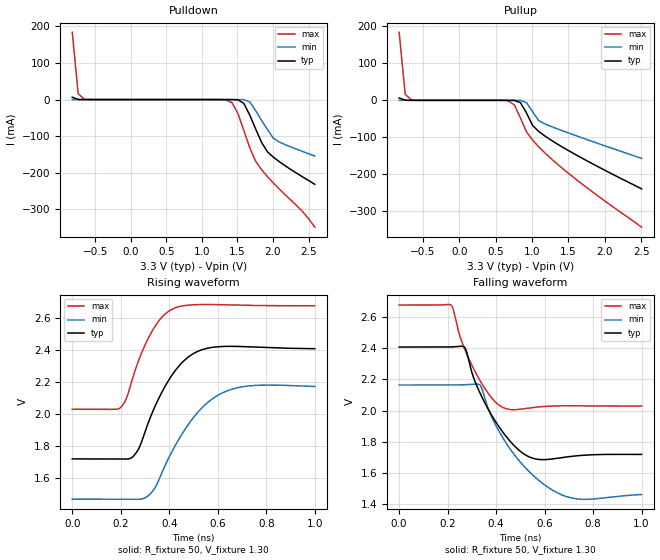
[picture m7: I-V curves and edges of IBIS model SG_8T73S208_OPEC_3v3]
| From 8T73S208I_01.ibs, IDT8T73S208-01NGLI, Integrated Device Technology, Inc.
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[Model] SG_8T73S208_OPEC_3v3
Model_type   Output_ECL
Polarity   Non-Inverting
|   typ   min   max
C_comp   2pF   1.5pF   2.5pF
Vmeas = 2.06V
Rref = 50
Cref = 0
Vref = 1.3V
|   typ   min   max
[Voltage range]   3.3V   3.135V   3.465V
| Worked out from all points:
|   rising waveform, R_fixture 50, V_fixture 1.30: 20-80 % time 131ps typ, 167ps min, 104ps max; typ from 1.72 V to 2.41 V
|   falling waveform, R_fixture 50, V_fixture 1.30: 20-80 % time 135ps typ, 176ps min, 108ps max; typ from 2.41 V to 1.72 V
[Pulldown]
|Voltage   I (typ)   I (min)   I (max)
|Note, modeling breaks down at 250mA and above.  This is well beyond the functional   |
|operating range of the device.  Should this scenario occur, catastrophic failure and   |
|possible damage to the device and/or board is of higher concern than the I-V curve   |
|behavior.  The IBIS checker will flag currents in excess of 10A with warnings.  Lines   |
|with currents in excess of 0.35 A have been commented out.  The points still remain|
|available to the user if the user desires to use them.   |
|-3.04000e+00   3.84320e+08   5.02796e+08   2.78359e+08
|-2.78000e+00   3.25714e+08   4.27850e+08   2.34472e+08
|-2.52000e+00   2.67107e+08   3.52905e+08   1.90585e+08
|-2.26000e+00   2.08500e+08   2.77959e+08   1.46698e+08
|-2.00000e+00   1.49893e+08   2.03013e+08   1.02811e+08
|-1.99000e+00   1.47639e+08   2.00131e+08   1.01123e+08
|-1.90678e+00   1.28880e+08   1.76142e+08   8.70758e+07
|-1.82356e+00   1.10121e+08   1.52153e+08   7.30282e+07
|-1.74033e+00   9.13618e+07   1.28164e+08   5.89806e+07
|-1.65711e+00   7.26027e+07   1.04175e+08   4.49331e+07
|-1.57389e+00   5.38435e+07   8.01855e+07   3.08855e+07
|-1.49067e+00   3.50844e+07   5.61965e+07   1.68379e+07
|-1.40744e+00   1.63252e+07   3.22075e+07   3.44928e+06
|-1.32422e+00   1.39944e+06   8.21842e+06   3.05002e+05
|-1.24100e+00   5.48675e+04   1.39917e+05   2.69841e+04
|-1.15778e+00   2.16294e+03   2.23572e+03   2.39776e+03
|-1.07456e+00   9.10504e+01   4.03625e+01   2.19447e+02
|-9.91333e-01   4.16516e+00   7.07425e-01   2.24205e+01
|-9.08111e-01   1.63247e-01   1.12381e-02   2.07885e+00
-824.9mV  6.398mA    178.5uA    183.8mA
-741.7mV  250.8uA    2.836uA    16.25mA
-658.4mV  9.828uA    45.07nA    1.437mA
1.256V    -48.99nA   -26.95pA   -86.69uA
1.422V    -28.87uA   -51.73nA   -8.139mA
1.505V    -675.9uA   -3.061uA   -37.65mA
1.589V    -10.23mA   -178.4uA   -83.91mA
1.672V    -41.96mA   -6.141mA   -131.5mA
1.755V    -80.08mA   -29.91mA   -168.3mA
1.921V    -142.8mA   -82.08mA   -210.6mA
2.005V    -157.3mA   -105.4mA   -228mA
2.587V    -231.4mA   -154.2mA   -348.7mA
| 2.67044e+00   -2.41524e-01   -1.60336e-01   -3.73288e-01
| 2.75367e+00   -2.52751e-01   -1.66631e-01   -3.98898e-01
| 2.83689e+00   -2.65451e-01   -1.73020e-01   -4.24212e-01
| 2.92011e+00   -2.79209e-01   -1.79583e-01   -4.49830e-01
| 3.00333e+00   -2.93544e-01   -1.86399e-01   -4.74213e-01
| 3.08656e+00   -3.07724e-01   -1.93355e-01   -4.94882e-01
| 3.16978e+00   -3.22002e-01   -2.00371e-01   -5.14267e-01
| 3.25300e+00   -3.36250e-01   -2.07556e-01   -5.33445e-01
| 3.33622e+00   -3.50790e-01   -2.15122e-01   -5.52591e-01
| 3.41944e+00   -3.64214e-01   -2.22630e-01   -5.71683e-01
| 3.50267e+00   -3.76611e-01   -2.29517e-01   -5.90648e-01
| 3.58589e+00   -3.88349e-01   -2.35518e-01   -6.09407e-01
| 3.66911e+00   -3.99917e-01   -2.41393e-01   -6.27633e-01
| 3.75233e+00   -4.11365e-01   -2.47762e-01   -6.44990e-01
| 3.83556e+00   -4.22795e-01   -2.54787e-01   -6.61715e-01
| 3.91878e+00   -4.34231e-01   -2.62348e-01   -6.78105e-01
| 4.00200e+00   -4.45476e-01   -2.70694e-01   -6.94450e-01
| 4.08522e+00   -4.57292e-01   -2.96778e-01   -7.11369e-01
| 4.16844e+00   -4.85300e-01   -3.52090e-01   -7.34921e-01
| 4.25167e+00   -5.33887e-01   -4.07605e-01   -7.78590e-01
| 4.33489e+00   -5.82604e-01   -4.63296e-01   -8.23081e-01
| 4.41811e+00   -6.31415e-01   -5.19140e-01   -8.67469e-01
| 4.50133e+00   -6.80294e-01   -5.75117e-01   -9.11758e-01
| 4.58456e+00   -7.29224e-01   -6.31213e-01   -9.55953e-01
| 4.66778e+00   -7.78192e-01   -6.87415e-01   -1.00006e+00
| 4.75100e+00   -8.27189e-01   -7.43713e-01   -1.04409e+00
| 4.83422e+00   -8.76208e-01   -8.00099e-01   -1.08807e+00
| 4.91744e+00   -9.25247e-01   -8.56569e-01   -1.13203e+00
| 5.00067e+00   -9.74313e-01   -9.13130e-01   -1.17598e+00
| 5.08389e+00   -1.02342e+00   -9.69776e-01   -1.21988e+00
| 5.16711e+00   -1.07255e+00   -1.02650e+00   -1.26381e+00
| 5.25033e+00   -1.12176e+00   -1.08332e+00   -1.30859e+00
| 5.33356e+00   -1.17164e+00   -1.14140e+00   -1.35828e+00
| 5.41678e+00   -1.22659e+00   -1.20480e+00   -1.40940e+00
| 5.50000e+00   -1.28295e+00   -1.26925e+00   -1.46042e+00
| 5.51000e+00   -1.28972e+00   -1.27702e+00   -1.46654e+00
| 5.72800e+00   -1.43794e+00   -1.44641e+00   -1.59960e+00
| 5.94600e+00   -1.59631e+00   -1.61583e+00   -1.73573e+00
| 6.16400e+00   -1.75745e+00   -1.78535e+00   -1.88508e+00
| 6.38200e+00   -1.91661e+00   -1.95502e+00   -2.03321e+00
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[Pullup]
|Voltage   I (typ)   I (min)   I (max)
|Note, modeling breaks down at 250mA and above.  This is well beyond the functional   |
|operating range of the device.  Should this scenario occur, catastrophic failure and   |
|possible damage to the device and/or board is of higher concern than the I-V curve   |
|behavior.  The IBIS checker will flag currents in excess of 10A with warnings.  Lines   |
|with currents in excess of 0.35 A have been commented out.  The points still remain|
|available to the user if the user desires to use them.   |
|-3.04000e+00   3.84320e+08   5.02796e+08   2.78359e+08
|-2.78000e+00   3.25714e+08   4.27850e+08   2.34472e+08
|-2.52000e+00   2.67107e+08   3.52905e+08   1.90585e+08
|-2.26000e+00   2.08500e+08   2.77959e+08   1.46698e+08
|-2.00000e+00   1.49893e+08   2.03013e+08   1.02811e+08
|-1.99000e+00   1.47639e+08   2.00131e+08   1.01123e+08
|-1.90678e+00   1.28880e+08   1.76142e+08   8.70758e+07
|-1.82356e+00   1.10121e+08   1.52153e+08   7.30282e+07
|-1.74033e+00   9.13618e+07   1.28164e+08   5.89806e+07
|-1.65711e+00   7.26027e+07   1.04175e+08   4.49331e+07
|-1.57389e+00   5.38435e+07   8.01855e+07   3.08855e+07
|-1.49067e+00   3.50844e+07   5.61965e+07   1.68379e+07
|-1.40744e+00   1.63252e+07   3.22075e+07   3.44928e+06
|-1.32422e+00   1.39944e+06   8.21842e+06   3.05002e+05
|-1.24100e+00   5.48675e+04   1.39917e+05   2.69841e+04
|-1.15778e+00   2.16294e+03   2.23572e+03   2.39776e+03
|-1.07456e+00   9.10504e+01   4.03625e+01   2.19447e+02
|-9.91333e-01   4.16516e+00   7.07425e-01   2.24205e+01
|-9.08111e-01   1.63247e-01   1.12381e-02   2.07885e+00
-824.9mV  6.398mA    178.5uA    183.8mA
-741.7mV  250.8uA    2.836uA    16.25mA
-658.4mV  9.828uA    45.07nA    1.437mA
673.1mV   -14.29uA   -53.29nA   -1.52mA
756.3mV   -340uA     -3.154uA   -12.35mA
839.6mV   -6.206mA   -183.8uA   -47.35mA
922.8mV   -33.74mA   -6.254mA   -85.15mA
1.006V    -67.53mA   -30.09mA   -107.4mA
1.089V    -83.8mA    -54.53mA   -125.3mA
1.172V    -95.98mA   -63.28mA   -141.5mA
1.672V    -154.7mA   -100.3mA   -224mA
2.504V    -239.1mA   -156.9mA   -342.7mA
| 2.58722e+00   -2.47244e-01   -1.62439e-01   -3.55238e-01
| 2.67044e+00   -2.55497e-01   -1.67965e-01   -3.69664e-01
| 2.75367e+00   -2.63903e-01   -1.73494e-01   -3.87482e-01
| 2.83689e+00   -2.72370e-01   -1.79082e-01   -4.08950e-01
| 2.92011e+00   -2.80902e-01   -1.84706e-01   -4.32860e-01
| 3.00333e+00   -2.90116e-01   -1.90329e-01   -4.57578e-01
| 3.08656e+00   -3.01259e-01   -1.95936e-01   -4.82435e-01
| 3.16978e+00   -3.14021e-01   -2.01551e-01   -5.06729e-01
| 3.25300e+00   -3.28024e-01   -2.07525e-01   -5.29945e-01
| 3.33622e+00   -3.42660e-01   -2.14086e-01   -5.52171e-01
| 3.41944e+00   -3.57227e-01   -2.20851e-01   -5.73066e-01
| 3.50267e+00   -3.71552e-01   -2.27604e-01   -5.92395e-01
| 3.58589e+00   -3.85312e-01   -2.34269e-01   -6.10638e-01
| 3.66911e+00   -3.97414e-01   -2.40591e-01   -6.28124e-01
| 3.75233e+00   -4.08570e-01   -2.47083e-01   -6.45029e-01
| 3.83556e+00   -4.19491e-01   -2.54178e-01   -6.61491e-01
| 3.91878e+00   -4.30565e-01   -2.61791e-01   -6.77703e-01
| 4.00200e+00   -4.41855e-01   -2.70182e-01   -6.93908e-01
| 4.08522e+00   -4.54060e-01   -2.96313e-01   -7.10701e-01
| 4.16844e+00   -4.82496e-01   -3.51673e-01   -7.34128e-01
| 4.25167e+00   -5.31421e-01   -4.07237e-01   -7.77667e-01
| 4.33489e+00   -5.80395e-01   -4.62980e-01   -8.22014e-01
| 4.41811e+00   -6.29408e-01   -5.18876e-01   -8.66242e-01
| 4.50133e+00   -6.78456e-01   -5.74907e-01   -9.10352e-01
| 4.58456e+00   -7.27534e-01   -6.31056e-01   -9.54351e-01
| 4.66778e+00   -7.76635e-01   -6.87308e-01   -9.98252e-01
| 4.75100e+00   -8.25758e-01   -7.43649e-01   -1.04209e+00
| 4.83422e+00   -8.74899e-01   -8.00069e-01   -1.08592e+00
| 4.91744e+00   -9.24061e-01   -8.56565e-01   -1.12983e+00
| 5.00067e+00   -9.73265e-01   -9.13141e-01   -1.17391e+00
| 5.08389e+00   -1.02254e+00   -9.69794e-01   -1.21817e+00
| 5.16711e+00   -1.07189e+00   -1.02652e+00   -1.26258e+00
| 5.25033e+00   -1.12131e+00   -1.08334e+00   -1.30783e+00
| 5.33356e+00   -1.17138e+00   -1.14140e+00   -1.35786e+00
| 5.41678e+00   -1.22647e+00   -1.20480e+00   -1.40918e+00
| 5.50000e+00   -1.28293e+00   -1.26924e+00   -1.46031e+00
| 5.51000e+00   -1.28970e+00   -1.27700e+00   -1.46644e+00
| 5.72800e+00   -1.43799e+00   -1.44639e+00   -1.59959e+00
| 5.94600e+00   -1.59631e+00   -1.61581e+00   -1.73572e+00
| 6.16400e+00   -1.75748e+00   -1.78536e+00   -1.88507e+00
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[Ramp]
|   typ   min   max
dV/dt_r   0.421/0.136n   0.427/0.171n   0.392/0.106n
dV/dt_f   0.434/0.147n   0.441/0.191n   0.403/0.115n
R_load =   50.0000
[Rising Waveform]
R_fixture = 50
V_fixture = 1.30   | VCC_typ - 2V
V_fixture_max = 1.465   | VCC_max - 2V
V_fixture_min = 1.135   | VCC_min - 2V
C_fixture = 0.0p
| Time   typ   min   max
0s        1.719V     1.468V     2.029V
193.2ps   1.718V     1.468V     2.033V
221.2ps   1.718V     1.468V     2.089V
248.2ps   1.731V     1.467V     2.218V
278.3ps   1.796V     1.468V     2.351V
331.3ps   2.013V     1.518V     2.521V
418.4ps   2.257V     1.785V     2.657V
521.5ps   2.392V     2.016V     2.681V
626.6ps   2.42V      2.136V     2.68V
1ns       2.406V     2.171V     2.674V
[Falling Waveform]
R_fixture = 50
V_fixture = 1.30   | VCC_typ - 2V
V_fixture_max = 1.465   | VCC_max - 2V
V_fixture_min = 1.135   | VCC_min - 2V
C_fixture = 0.0p
| Time   typ   min   max
0s        2.406V     2.163V     2.674V
213.2ps   2.406V     2.163V     2.674V
268.3ps   2.406V     2.164V     2.4V
335.3ps   2.106V     2.159V     2.186V
377.4ps   1.981V     1.973V     2.089V
432.4ps   1.852V     1.814V     2.016V
540.5ps   1.701V     1.603V     2.017V
675.7ps   1.7V       1.458V     2.03V
770.8ps   1.715V     1.433V     2.03V
1ns       1.719V     1.463V     2.028V
